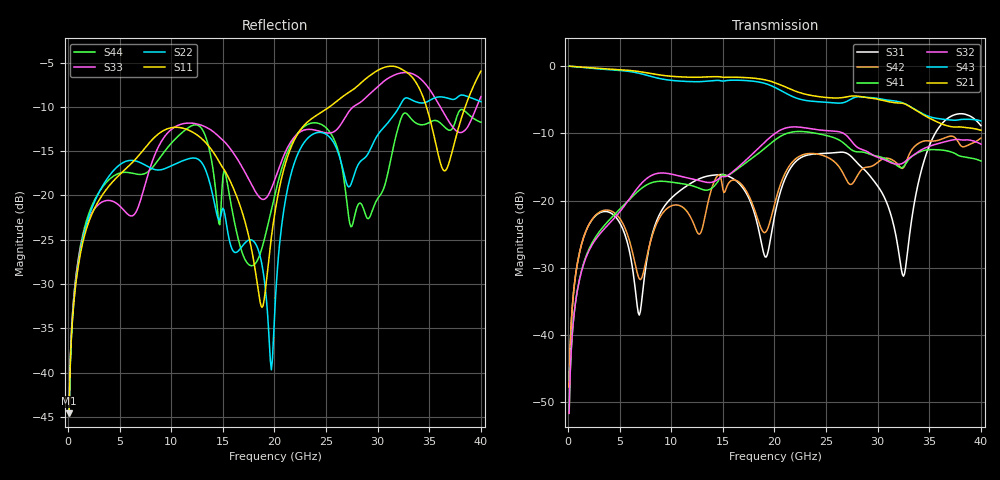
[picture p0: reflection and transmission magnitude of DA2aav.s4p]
! ADC12DJ2700AAV, ADC12DJ3200AAV, ADC08DJ3200AAV
! 144 pin AAV package
! Texas Instruments 4/21/2021
! Single-ended  S-parameters
! PORT#  PORT_NAME  NET_NAME
! PORT1:  DAxN.DIEBUMP DAxN
! PORT2:  DAxN.BGA  DAxN
! PORT3:  DAxP.DIEBUMP DAxP
! PORT4:  DAxP.BGA  DAxP
! Touchstone Ver. 1.0
! Number of ports is 4
# Hz	S	MA	R	50.000000
! SCATTERING PARAMETERS  :
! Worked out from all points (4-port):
!   400 points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, 100 MHz to 40 GHz, reference 50 ohm
!   strongest paths, dB at 100 MHz, 10.1 GHz, 20.1 GHz, 30.1 GHz, 40 GHz:
!     S21: 0.0, -1.5, -2.5, -5.0, -9.5
!     S43: 0.0, -2.1, -3.2, -4.8, -8.2
!     S32: -51.6, -16.1, -10.0, -13.6, -11.6
!     S41: -51.6, -17.3, -10.9, -13.4, -14.1
!     S42: -47.7, -20.7, -20.0, -14.2, -10.7
!     S31: -47.7, -19.5, -21.6, -18.1, -8.9
!   lowest |S11| = -44.6 dB at 100 MHz (marker M1), VSWR 1.01, Z = 50.3 + j0.527 ohm
!   |S11| at or under -10 dB: start of sweep to 25.33 GHz; 34.73 GHz to 38.48 GHz (3.753 GHz wide, 10.3 % of centre)
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1e8  0.005894 62.8  0.997 -1.9  0.004117 84.1  0.002621 -98.0
     0.997 -1.9  0.005911 61.7  0.00262 -98.0  0.004112 84.0
     0.004117 84.1  0.00262 -98.0  0.006119 65.3  0.9972 -1.8
     0.002621 -98.0  0.004112 84.0  0.9972 -1.8  0.006116 64.6
2.1e9  0.07333 52.9  0.9716 -36.6  0.06776 45.0  0.0448 -144.4
       0.9716 -36.6  0.07866 26.5  0.04351 -142.8  0.06798 43.7
       0.06776 45.0  0.04351 -142.8  0.07581 44.0  0.9649 -35.4
       0.0448 -144.4  0.06798 43.7  0.9649 -35.4  0.08166 31.4
1.03e10  0.2424 -18.6  0.8356 -171.6  0.1094 59.1  0.136 52.9
         0.8356 -171.6  0.1499 -100.9  0.1554 62.3  0.0926 25.4
         0.1094 59.1  0.1554 62.3  0.2426 7.2  0.7782 -162.8
         0.136 52.9  0.0926 25.4  0.7782 -162.8  0.2059 -78.5
1.97e10  0.05824 34.7  0.7675 28.8  0.05689 66.6  0.2689 -85.7
         0.7675 28.8  0.01037 112.6  0.3005 -69.4  0.07611 25.7
         0.05689 66.6  0.3005 -69.4  0.1093 137.5  0.7127 47.7
         0.2689 -85.7  0.07611 25.7  0.7127 47.7  0.08331 52.6
2.3e10  0.2534 -0.6  0.6172 -23.9  0.2156 34.6  0.3245 -164.9
        0.6172 -23.9  0.2035 -54.6  0.3467 -147.8  0.2217 -29.3
        0.2156 34.6  0.3467 -147.8  0.235 29.5  0.555 2.2
        0.3245 -164.9  0.2217 -29.3  0.555 2.2  0.2477 -44.5
3.25e10  0.5088 -106.6  0.5269 179.3  0.02739 -147.2  0.1784 33.0
         0.5269 179.3  0.3475 -88.2  0.1909 58.4  0.1754 133.5
         0.02739 -147.2  0.1909 58.4  0.4937 -61.3  0.53 -144.8
         0.1784 33.0  0.1754 133.5  0.53 -144.8  0.2891 -57.1
4e10  0.5032 -25.6  0.3331 61.4  0.3602 -40.8  0.1968 -119.8
      0.3331 61.4  0.3385 -130.8  0.263 -92.6  0.291 67.1
      0.3602 -40.8  0.263 -92.6  0.3614 69.8  0.3905 100.2
      0.1968 -119.8  0.291 67.1  0.3905 100.2  0.259 -95.3
